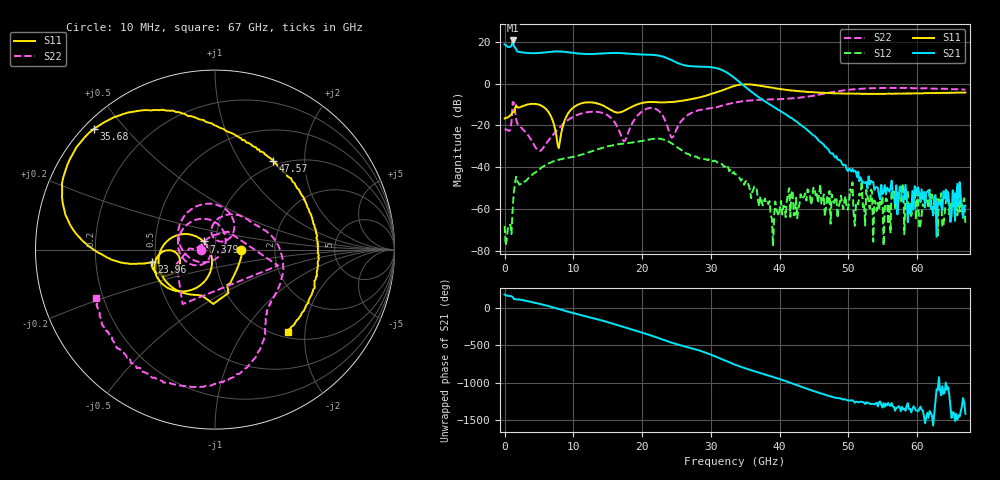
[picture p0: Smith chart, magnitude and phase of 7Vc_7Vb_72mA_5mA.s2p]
! MARKI MICROWAVE INC.
! Date:  05/05/2020
! Model Number:  APM-7099CH
! Description:  2-port Small Signal S-parameter data for APM-7099CH
! Frequency Range:  10 MHz to 67 GHz
! Port Configuration:  PORT 1: Input
!  PORT 2: Output
! Bias Condition: Vc = +7V, Vb = +7V
! APM-7099CH s2p files are only valid for small signal conditions (below -5 dBm input power)
!S2P File: Measurements: Mag<S11> Ang<S11>, Mag<S21> Ang<S21>, Mag<S12> Ang<S12>, Mag<S22> Ang<S22>!row 1
# Hz S  dB  R 50
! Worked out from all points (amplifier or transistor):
!   401 points, 10 MHz to 67 GHz, reference 50 ohm
!   highest |S21| = 20.6 dB at 1.182 GHz (marker M1)
!   |S21| within 3 dB of that: start of sweep to 472.9 MHz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
!   unconditionally stable (mu >= 1): start of sweep to end of sweep
!   at 11.06 GHz: K = 4.24, MAG = 14.9 dB, |S12| = -34.1 dB
!   at 33.51 GHz: K = 9.96, MAG = 9.9 dB, |S12| = -43.3 dB
!   at 67 GHz: K = 284175.80, MAG = -53.2 dB, |S12| = -67.1 dB
!   S11 on the Smith chart (normalised r, x): 10 MHz: 1.35, +0.00; 7.379 GHz: 0.88, +0.08; 23.96 GHz: 0.48, -0.08; 35.68 GHz: 0.03, +0.41; 47.57 GHz: 0.93, +1.41; 67 GHz: 1.10, -1.63
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1e7  -16.63 0.2  18.70 178.5  -67.87 -81.0  -22.09 -177.1
1.182325e9  -13.72 -65.7  20.57 145.9  -59.89 78.2  -8.82 -14.2
1.68475e9  -10.38 -91.8  16.37 113.0  -44.47 -80.8  -16.90 177.4
4.866775e9  -9.94 -170.7  14.56 59.6  -41.21 -175.2  -31.91 -179.4
7.3789e9  -22.15 144.5  15.32 -1.1  -36.79 124.2  -23.19 -123.8
9.3886e9  -13.55 -111.7  14.88 -54.3  -35.32 81.2  -17.04 -141.4
1.123082e10  -9.37 -141.3  14.21 -98.4  -33.88 48.5  -14.22 -172.0
1.47478e10  -11.25 -178.9  14.47 177.0  -30.21 -23.1  -14.70 110.9
1.60876e10  -13.65 -171.7  14.61 140.3  -29.24 -54.4  -18.88 65.8
1.759488e10  -12.64 -152.6  14.40 97.9  -28.55 -90.3  -26.72 -70.5
2.027448e10  -9.08 -158.7  13.82 23.4  -27.19 -154.6  -12.68 151.3
2.245165e10  -8.96 -168.9  13.32 -44.3  -26.33 140.1  -13.09 69.2
2.395892e10  -8.93 -168.9  11.70 -93.8  -27.91 89.0  -23.35 42.4
2.697348e10  -7.56 -169.2  8.31 -171.2  -34.19 24.3  -14.32 77.0
2.982055e10  -5.22 -173.1  7.90 103.0  -36.91 -25.0  -11.85 36.7
3.166278e10  -3.24 179.3  6.40 33.1  -38.59 -67.2  -10.54 21.1
3.3505e10  -1.03 163.0  2.49 -37.0  -43.28 -104.8  -9.02 3.8
3.568218e10  -0.43 134.9  -3.37 -106.0  -50.93 -146.5  -8.03 -16.3
4.472582e10  -4.11 72.4  -24.27 -21.7  -55.36 -34.3  -5.91 -56.3
4.75729e10  -4.59 56.8  -33.36 -104.9  -52.87 -47.4  -4.19 -67.0
5.594665e10  -4.80 8.0  -51.66 142.9  -57.39 -54.2  -2.06 -111.8
6.7e10  -4.25 -48.6  -58.31 27.8  -67.09 38.1  -2.92 -157.9
